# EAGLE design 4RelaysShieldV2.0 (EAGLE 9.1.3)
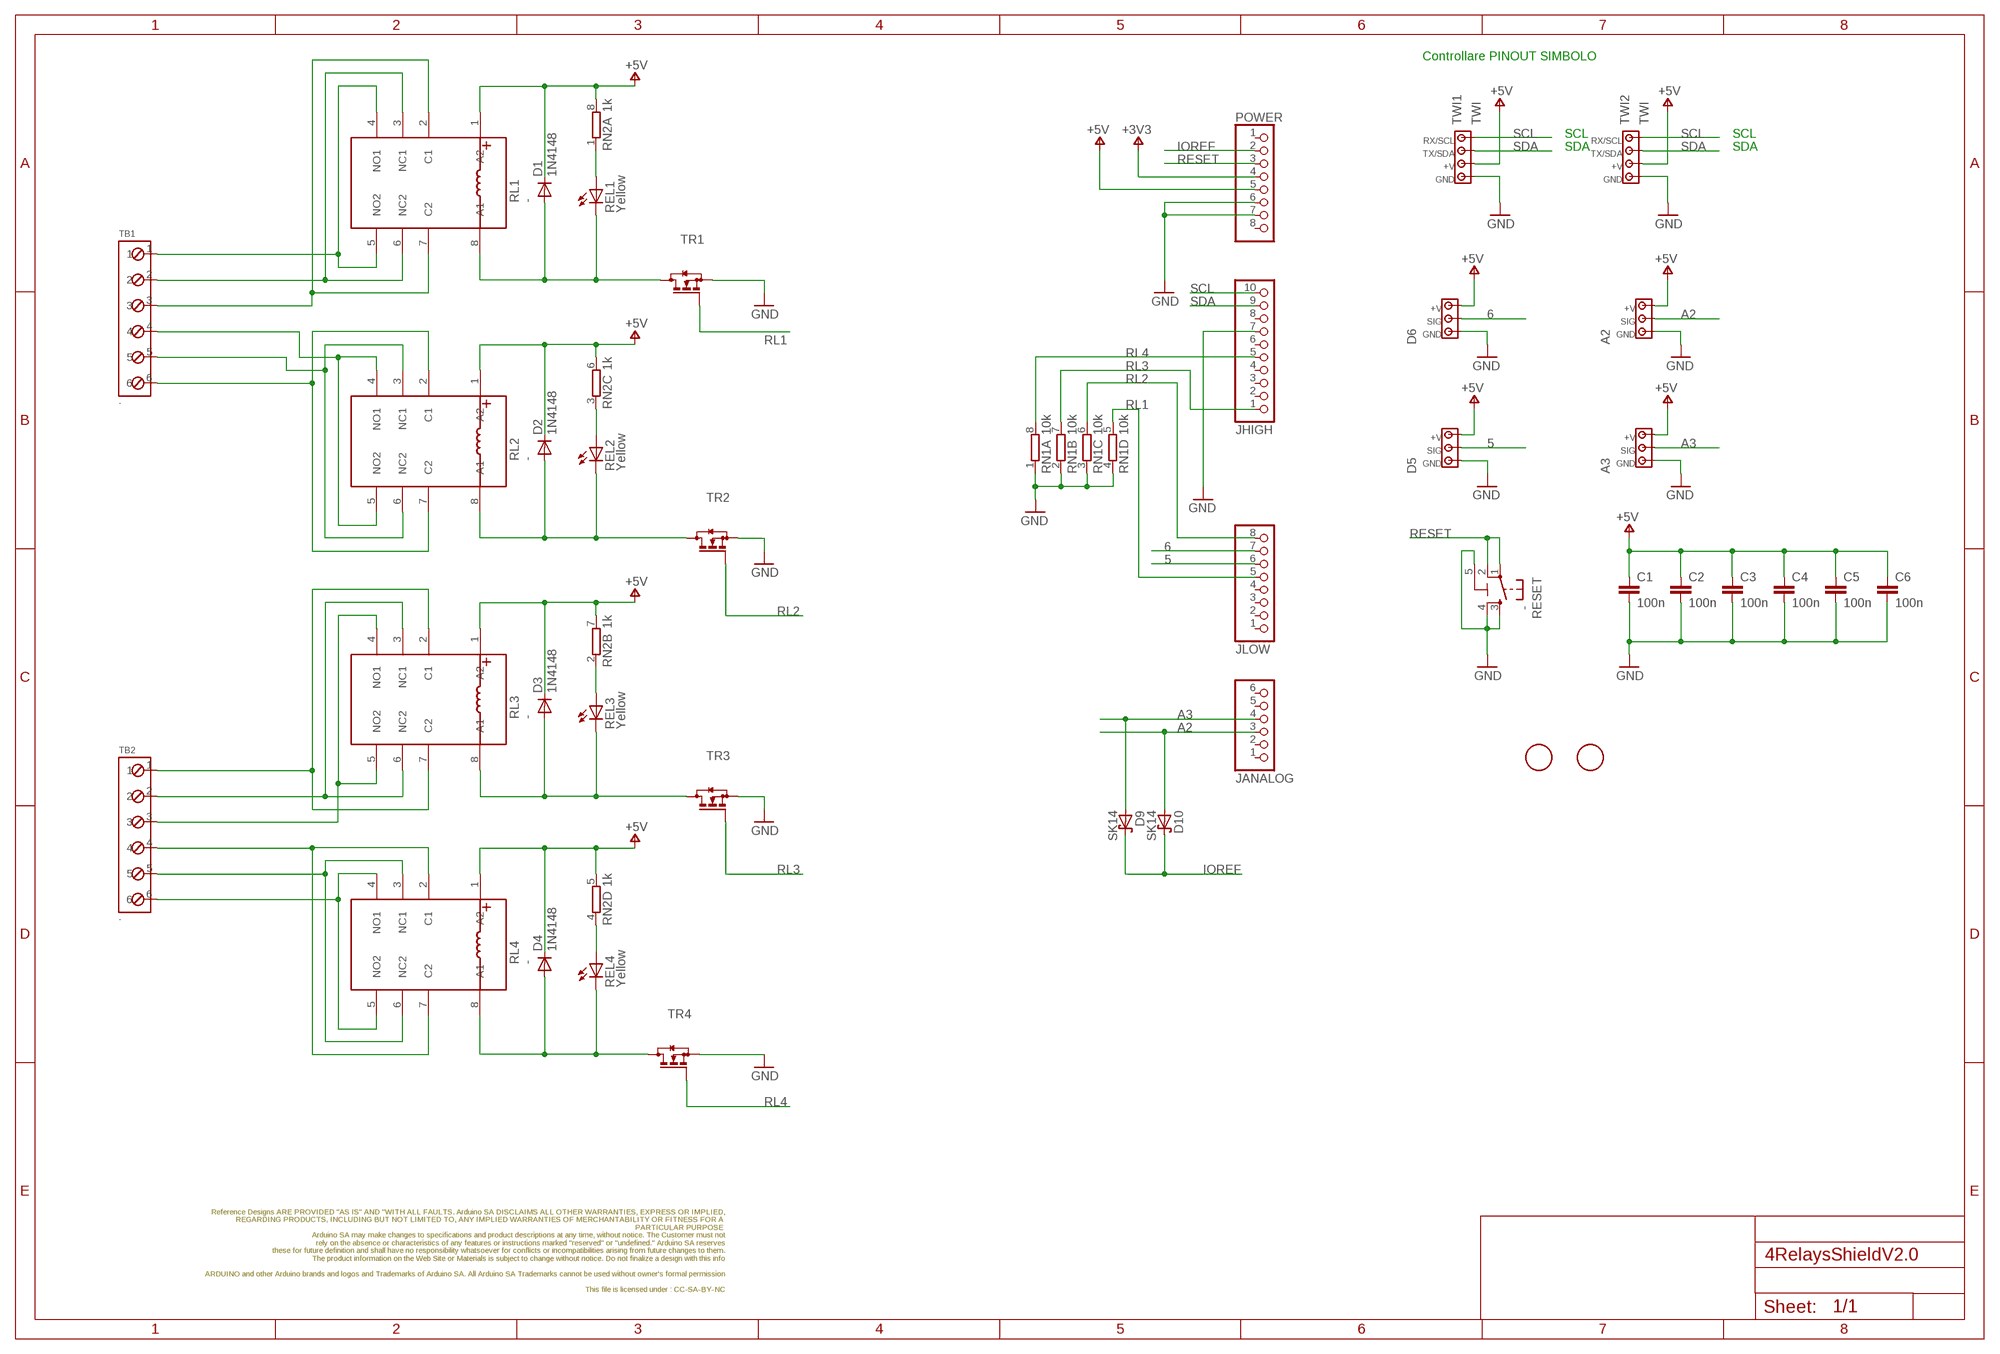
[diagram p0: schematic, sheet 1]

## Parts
A2  -  MODULINO-3-IN  [MODULINO-3]
A3  -  MODULINO-3-IN  [MODULINO-3]
C1  100n  C-100NF-0603  [0603-1608X90N]
C2  100n  C-100NF-0603  [0603-1608X90N]
C3  100n  C-100NF-0603  [0603-1608X90N]
C4  100n  C-100NF-0603  [0603-1608X90N]
C5  100n  C-100NF-0603  [0603-1608X90N]
C6  100n  C-100NF-0603  [0603-1608X90N]
D1  1N4148  DIODE-SOD123  [SOD123]
D2  1N4148  DIODE-SOD123  [SOD123]
D3  1N4148  DIODE-SOD123  [SOD123]
D4  1N4148  DIODE-SOD123  [SOD123]
D5  OUT  MODULINO-3-OUT  [MODULINO-3]
D6  OUT  MODULINO-3-OUT  [MODULINO-3]
D9  SK14  D_SCHOTTKY-SMB-SMB  [SMB_DO214AA]
D10  SK14  D_SCHOTTKY-SMB-SMB  [SMB_DO214AA]
FID2  DNP  FIDUCIAL-2MM  [FD-1-2]
FID3  DNP  FIDUCIAL-2MM  [FD-1-2]
FRAME1  A3-FRAMEONLY  [FRAME-NO-BAN-FRAMEONLY]
FRAME2  TEXTTEXT_BRDSCH  [FRAME]
JANALOG  Analog  PINHD-1X06TH  [1X06-TH]
JHIGH  Digital  PINHD-1X10TH  [1X10]
JLOW  Digital  PINHD-1X08-DIGITALTH  [1X08]
POWER  Power  PINHD-1X08-POWERTH  [1X08]
REL1  Yellow  0044_KPT-2012YC  [CHIPLED_0805]
REL2  Yellow  0044_KPT-2012YC  [CHIPLED_0805]
REL3  Yellow  0044_KPT-2012YC  [CHIPLED_0805]
REL4  Yellow  0044_KPT-2012YC  [CHIPLED_0805]
RESET  -  TACTILE2  [TS42]
RL1  -  RELAY-5  [RELE'-30SSERIES-DIL-2X]
RL2  -  RELAY-5  [RELE'-30SSERIES-DIL-2X]
RL3  -  RELAY-5  [RELE'-30SSERIES-DIL-2X]
RL4  -  RELAY-5  [RELE'-30SSERIES-DIL-2X]
RN1  10k  4R-N-10KCAY16  [CAY16]
RN2  1k  4R-N-1KCAY16  [CAY16]
TB1  -  0698_MRB316-3,81-V-BL  [MRB316-3,81-V-BL]
TB2  -  0698_MRB316-3,81-V-BL  [MRB316-3,81-V-BL]
TR1  2N7002  2N7002T-SOT23-SOT23  [SOT23]
TR2  2N7002  2N7002T-SOT23-SOT23  [SOT23]
TR3  2N7002  2N7002T-SOT23-SOT23  [SOT23]
TR4  2N7002  2N7002T-SOT23-SOT23  [SOT23]
TWI1  TWI  MODULINO-4-TWI  [MODULINO-4]
TWI2  TWI  MODULINO-4-TWI  [MODULINO-4]

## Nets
5: D5.2 JLOW.6
6: D6.2 JLOW.7
+3V3 [power]: POWER.4
+5V [power]: A2.1 A3.1 C1.1 C2.1 C3.1 C4.1 C5.1 C6.1 D1.C D2.C D3.C D4.C D5.1 D6.1 POWER.5 RL1.1(A2) RL2.1(A2) RL3.1(A2) RL4.1(A2) RN2.5 RN2.6 RN2.7 RN2.8 TWI1.3 TWI2.3
A2: A2.2 D10.A JANALOG.3
A3: A3.2 D9.A JANALOG.4
GND [power]: A2.3 A3.3 C1.2 C2.2 C3.2 C4.2 C5.2 C6.2 D5.3 D6.3 JHIGH.7 POWER.6 POWER.7 RESET.3 RESET.4 RESET.5(5-GND) RN1.1 RN1.2 RN1.3 RN1.4 TR1.2(S) TR2.2(S) TR3.2(S) TR4.2(S) TWI1.4 TWI2.4
IOREF: D9.C D10.C POWER.2
N$1: REL1.A RN2.1
N$2: REL2.A RN2.3
N$3: REL3.A RN2.2
N$4: REL4.A RN2.4
N$14: D1.A REL1.C RL1.8(A1) TR1.3(D)
N$16: D2.A REL2.C RL2.8(A1) TR2.3(D)
N$18: D3.A REL3.C RL3.8(A1) TR3.3(D)
N$20: D4.A REL4.C RL4.8(A1) TR4.3(D)
REL1_COM [RelayOut]: RL1.2(C1) RL1.7(C2) TB1.3
REL1_NC [RelayOut]: RL1.3(NC1) RL1.6(NC2) TB1.2
REL1_NO [RelayOut]: RL1.4(NO1) RL1.5(NO2) TB1.1
REL2_COM [RelayOut]: RL2.2(C1) RL2.7(C2) TB1.6
REL2_NC [RelayOut]: RL2.3(NC1) RL2.6(NC2) TB1.5
REL2_NO [RelayOut]: RL2.4(NO1) RL2.5(NO2) TB1.4
REL3_COM [RelayOut]: RL3.2(C1) RL3.7(C2) TB2.1
REL3_NC [RelayOut]: RL3.3(NC1) RL3.6(NC2) TB2.2
REL3_NO [RelayOut]: RL3.4(NO1) RL3.5(NO2) TB2.3
REL4_COM [RelayOut]: RL4.2(C1) RL4.7(C2) TB2.4
REL4_NC [RelayOut]: RL4.3(NC1) RL4.6(NC2) TB2.5
REL4_NO [RelayOut]: RL4.4(NO1) RL4.5(NO2) TB2.6
RESET: POWER.3 RESET.1 RESET.2
RL1: JLOW.5 RN1.5 TR1.1(G)
RL2: JLOW.8 RN1.6 TR2.1(G)
RL3: JHIGH.1 RN1.7 TR3.1(G)
RL4: JHIGH.5 RN1.8 TR4.1(G)
SCL: JHIGH.10 TWI1.1 TWI2.1
SDA: JHIGH.9 TWI1.2 TWI2.2
Unconnected: JANALOG.1 JANALOG.2 JANALOG.5 JANALOG.6 JHIGH.2 JHIGH.3 JHIGH.4 JHIGH.6 JHIGH.8 JLOW.1 JLOW.2 JLOW.3 JLOW.4 POWER.1 POWER.8

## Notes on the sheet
- Controllare PINOUT SIMBOLO
- SCL | SCL
- SDA | SDA

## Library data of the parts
A2 A3 = Arduino-connectors:MODULINO-3: Modulino 4 connector; CODE-BCE: SP1695; CODE-BCMI: 1695; CODE-TK2: -; DATASHEET: -; DISTRIBUTOR-LINK: -; DISTRIBUTOR-PN: -; MANUFACTURER: -; MANUFACTURER-PN: -
C1-C6 = Arduino-rcl:C: SMD Capacitor; CODE-ARDUINO: -; DATASHEET: http://search.murata.co.jp/Ceramy/image/img/A01X/G101/ENG/GRM188R71C104KA01-01.pdf; DISTRIBUTOR-LINK: https://www.digikey.com/product-detail/en/murata-electronics-north-america/GRM188R71C104KA01D/490-1532-1-ND/587771; DISTRIBUTOR-PN: 490-1532-2-ND; MANUFACTURER: Murata; MANUFACTURER-PN: GRM188R71C104KA01D; NOTE: -
D1-D4 = Arduino-diodes:DIODE: FAST SMALL SIGNAL DIODES SMD 200mA 100V SOD123; CODE-BCE: SP0234; CODE-BCMI: 0234; CODE-TK2: -; DATASHEET: http://www.mccsemi.com/up_pdf/1N4148WX(SOD323).pdf; DISTRIBUTOR-LINK: https://www.digikey.com/product-detail/it/micro-commercial-co/1N4148WX-TP/1N4148WXTPMSCT-ND/717312; DISTRIBUTOR-PN: 1N4148WXTPMSCT-ND; MANUFACTURER: Micro Commercial Co; MANUFACTURER-PN: 1N4148WX-TP
D5 D6 = Arduino-connectors:MODULINO-3: Modulino 4 connector; CODE-BCE: SP1696; CODE-BCMI: 1696; CODE-TK2: -; DATASHEET: -; DISTRIBUTOR-LINK: -; DISTRIBUTOR-PN: -; MANUFACTURER: -; MANUFACTURER-PN: -
D9 D10 = Arduino-diodes:D_SCHOTTKY: Schottky Diodes; CODE-ARDUINO: 0234; DATASHEET: http://www.mccsemi.com/up_pdf/SK12-L~SK110-L(DO-214AA).PDF; DISTRIBUTOR-LINK: https://www.digikey.com/product-detail/it/micro-commercial-co/SK14-LTP/SK14-LTPMSCT-ND/2642062; DISTRIBUTOR-PN: SK14-LTPMSCT-ND; MANUFACTURER: Micro Commercial Co; MANUFACTURER-PN: SK14-LTP
FID2 FID3 = Arduino-utility:FIDUCIAL: Fiducial mount; CODE-ARDUINO: DNP; DATASHEET: DNP; DISTRIBUTOR-LINK: DNP; DISTRIBUTOR-PN: DNP; MANUFACTURER: DNP; MANUFACTURER-PN: DNP
FRAME1 = Arduino-utility:A3-FRAMEONLY: Schematic frame
FRAME2 = Arduino-utility:TEXT: TEXT
JANALOG = Arduino-connectors:PINHD-1X06: PIN HEADER; CODE-ARDUINO: 3649; DATASHEET: -; DISTRIBUTOR-LINK: -; DISTRIBUTOR-PN: -; MANUFACTURER: -; MANUFACTURER-PN: FH254-106DF085149V
JHIGH = Arduino-connectors:PINHD-1X10: PIN HEADER; CODE-ARDUINO: 3648; DATASHEET: -; DISTRIBUTOR-LINK: -; DISTRIBUTOR-PN: -; MANUFACTURER: -; MANUFACTURER-PN: FH254-110DF085149V
JLOW = Arduino-connectors:PINHD-1X08: PIN HEADER; CODE-ARDUINO: 3648; DATASHEET: -; DISTRIBUTOR-LINK: -; DISTRIBUTOR-PN: -; MANUFACTURER: -; MANUFACTURER-PN: FH254-108DF085149V
POWER = Arduino-connectors:PINHD-1X08: PIN HEADER; CODE-ARDUINO: 3649; DATASHEET: -; DISTRIBUTOR-LINK: -; DISTRIBUTOR-PN: -; MANUFACTURER: -; MANUFACTURER-PN: FH254-108DF085149V
REL1-REL4 = Opto:0044_KPT-2012YC: LED YELLOW - SMD - 0805; MONTHLY_USAGE: _____; PART_NUMBER: KPT-2012YC; PRICE: _____; SUPPLIER: _____; TYPE: Opto
RESET = Arduino-pushbuttons:TACTILE2: Pushbutton; CODE-ARDUINO: 0946; DATASHEET: http://www.mouser.com/ds/2/418/NG_CD_1571636_C1-122399.pdf; DISTRIBUTOR-LINK: https://www.mouser.it/ProductDetail/TE-Connectivity/1571636-3/?qs=%2fha2pyFaduiys%2fNUBzym%252bcoSb9tuK3Sjuv54qjf0hQ0%3d; DISTRIBUTOR-PN: 506-1571636-3; MANUFACTURER: TE; MANUFACTURER-PN: 1571636-3
RL1-RL4 = Arduino-mechanical:RELAY-5: Relay 5V black Omron; CODE-BCE: SP0773; CODE-BCMI: 0773; CODE-TK2: -; DATASHEET: http://omronfs.omron.com/en_US/ecb/products/pdf/en-g5v_2.pdf; DISTRIBUTOR-LINK: https://www.digikey.com/product-detail/it/omron-electronics-inc-emc-div/G5V-2-H1-DC5/Z108-ND/277844; DISTRIBUTOR-PN: Z108-ND; MANUFACTURER: Omron; MANUFACTURER-PN: G5V-2-H1 DC5
RN1 = Arduino-rcl:4R-N: Array Chip Resistor Source: RS Component / Phycomp; CODE-ARDUINO: 0016; DATASHEET: http://www.bourns.com/docs/Product-Datasheets/CATCAY.pdf; DISTRIBUTOR-LINK: https://www.digikey.com/products/en?keywords=CAY16-103J4LFTR-ND; DISTRIBUTOR-PN: CAY16-103J4LFTR-ND; MANUFACTURER: Bourns Inc.; MANUFACTURER-PN: CAY16-103J4LF; RESTRICTIONS: NO
RN2 = Arduino-rcl:4R-N: Array Chip Resistor Source: RS Component / Phycomp; CODE-ARDUINO: 0005; DATASHEET: http://www.bourns.com/docs/Product-Datasheets/CATCAY.pdf; DISTRIBUTOR-LINK: https://www.digikey.com/product-detail/en/bourns-inc/CAY16-102J4LF/CAY16-102J4LFCT-ND/3437828; DISTRIBUTOR-PN: CAY16-102J4LFCT-ND; MANUFACTURER: Bourns Inc.; MANUFACTURER-PN: CAY16-102J4LF; RESTRICTIONS: NO
TB1 TB2 = Arduino-connectors:0698_MRB316-3,81-V-BL: Morsetto 6 poli h8,5mm Blue - EURO-BLOCK; CODE-BCE: SP0698; CODE-BCMI: 0698; CODE-TK2: -; DATASHEET: -; DISTRIBUTOR-LINK: -; DISTRIBUTOR-PN: -; MANUFACTURER: -; MANUFACTURER-PN: MRB316-3,81-V-BL
TR1-TR4 = Arduino-transistors:2N7002T: MOSFET N-CH 60V 115MA; CODE-ARDUINO: -; DATASHEET: http://www.mccsemi.com/up_pdf/2N7002(SOT-23).PDF; DISTRIBUTOR-LINK: https://www.digikey.com/product-detail/it/micro-commercial-co/2N7002-TP/2N7002-TPMSCT-ND/1960099; DISTRIBUTOR-PN: 2N7002-TPMSCT-ND; MANUFACTURER: Micro Commercial Co; MANUFACTURER-PN: 2N7002-TP
TWI1 TWI2 = Arduino-connectors:MODULINO-4: Modulino 4 connector; CODE-BCE: SP1693; CODE-BCMI: 1693; CODE-TK2: -; DATASHEET: -; DISTRIBUTOR-LINK: -; DISTRIBUTOR-PN: -; MANUFACTURER: -; MANUFACTURER-PN: -

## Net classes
0 default: width 0.254 mm, drill 0.61 mm, clearance 0.152 mm
1 power: width 0.305 mm, drill 0.61 mm, clearance 0.305 mm
2 VIN: width 0.305 mm, drill 0.61 mm, clearance 0.152 mm
3 RelayOut: width 1.27 mm, clearance 4 mm to class 0, clearance 4 mm to class 1, clearance 4 mm to class 2, clearance 1.27 mm

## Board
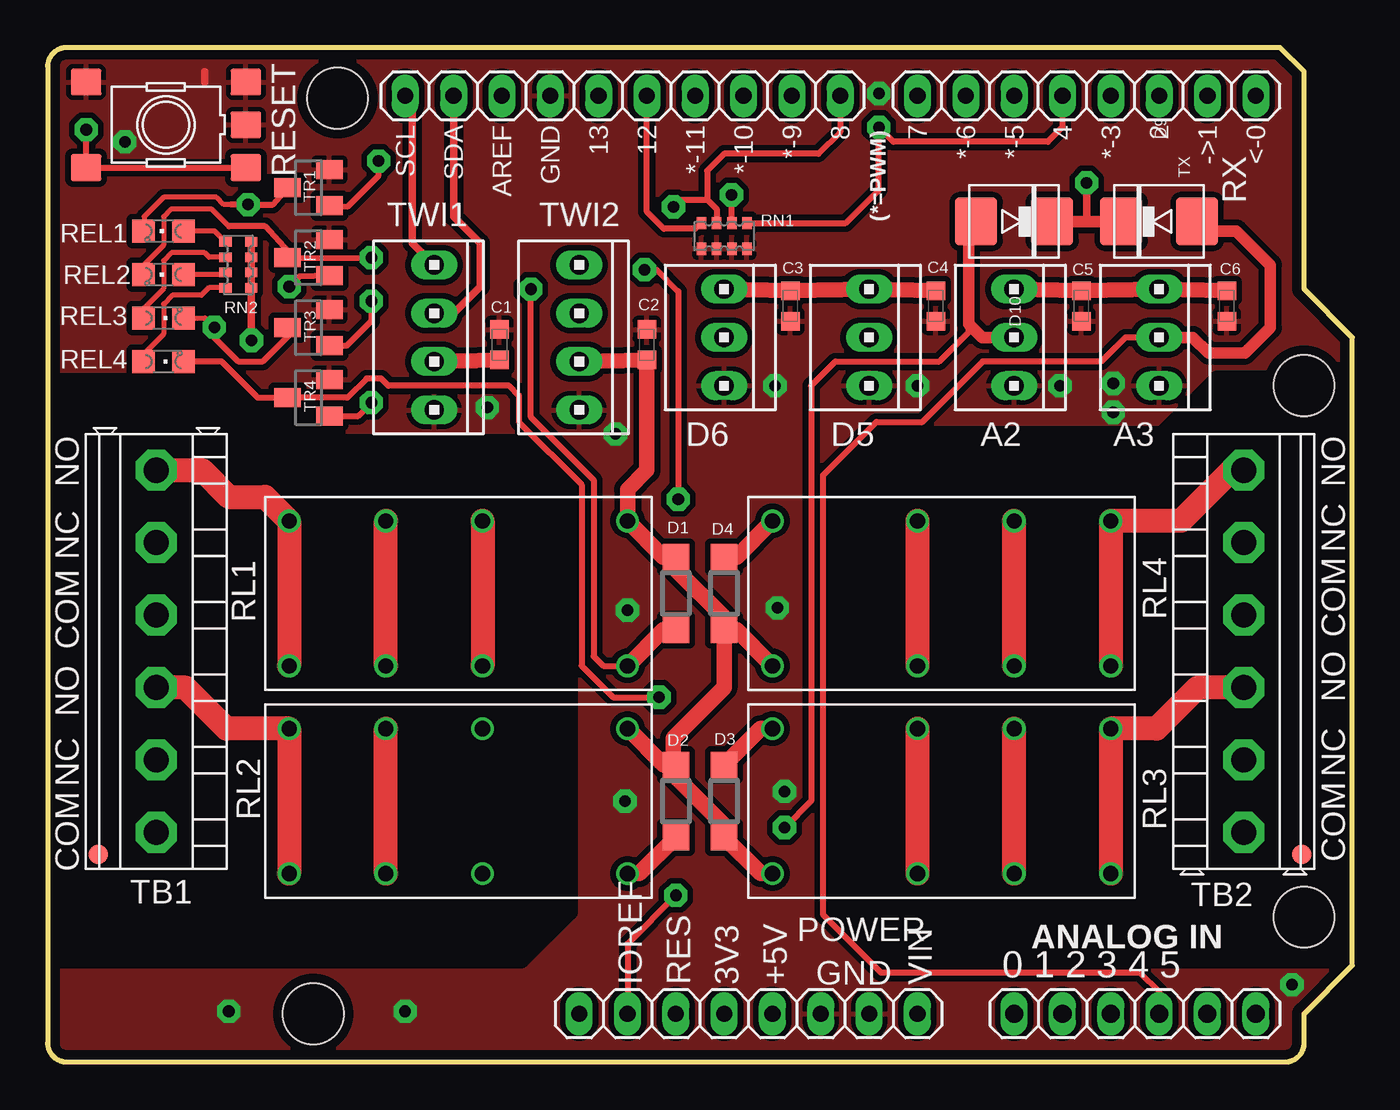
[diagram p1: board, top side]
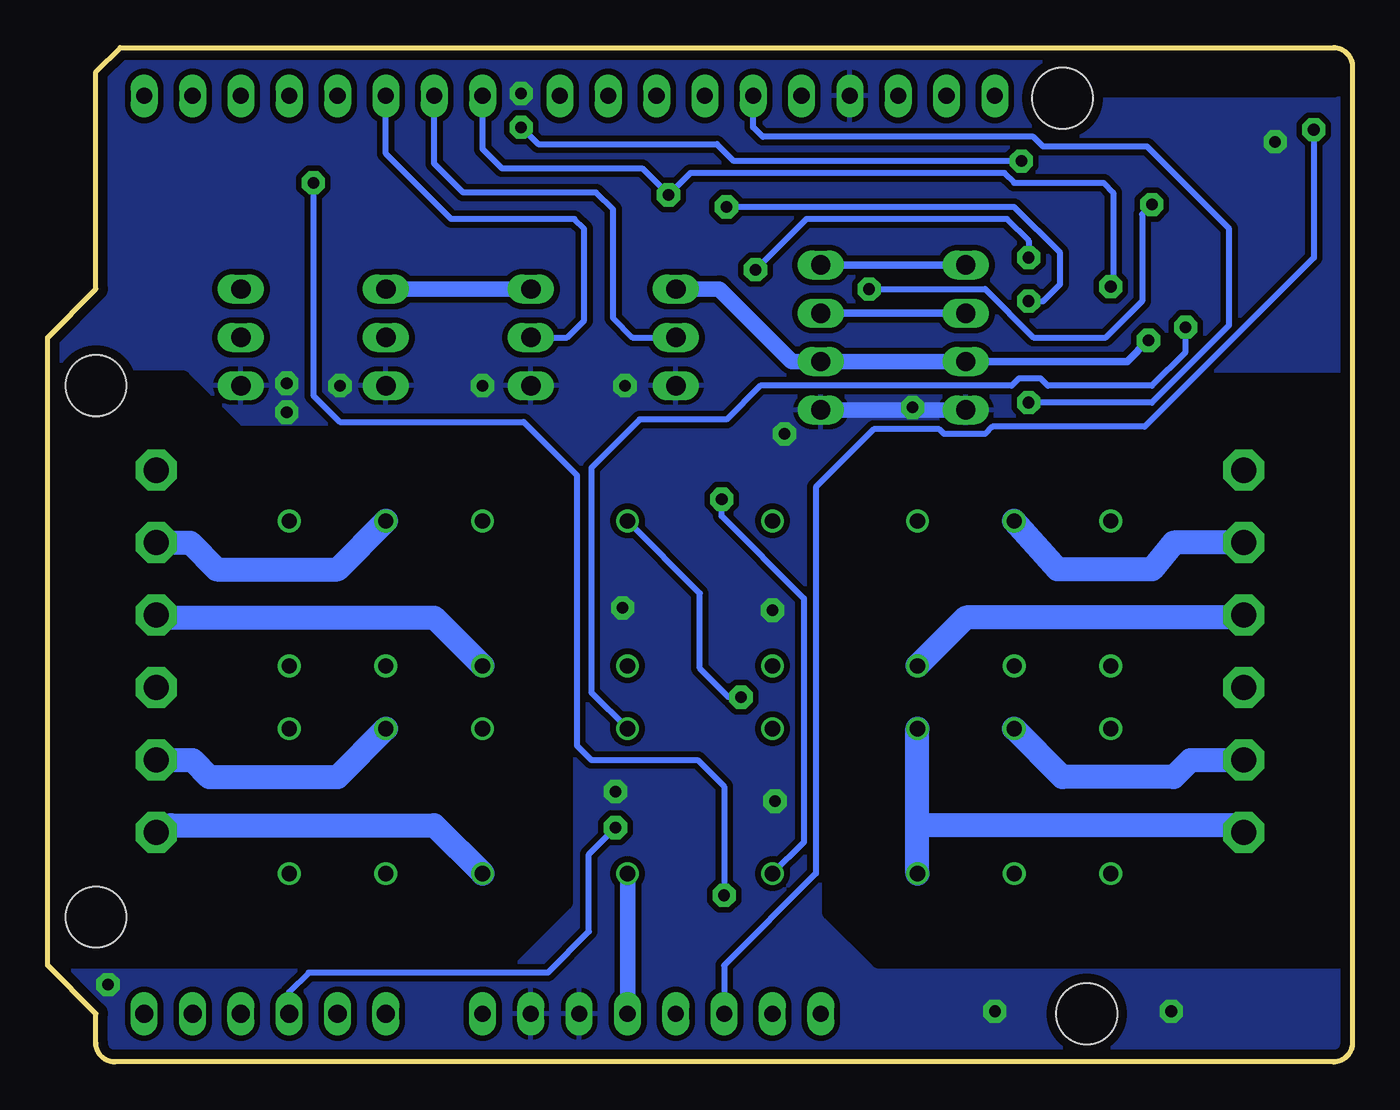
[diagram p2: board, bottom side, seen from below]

Size 68.58 x 53.34 mm. Coordinates in mm from the lower left corner, seen from the top.
Outline: 66.04,2.54 68.58,5.08 68.58,38.1 66.04,40.64 66.04,52.07 64.77,53.34 1,53.34 arc90 0,52.34 0,1 arc90 1,0 65.04,0 arc90 66.04,1 66.04,2.54
Copper layers (1*16): Top 0.035mm / dielectric 1.5mm / Bottom 0.035mm
Design rules "default *": minimum track width 10mil, minimum drill 10mil, track to track 12mil, track to pad 12mil, pad to pad 12mil, via to via 12mil, smd to smd 12mil, copper to edge 20mil, drill to drill 10mil, minimum pad ring 6mil, minimum via ring 12mil, stop-mask expansion 2mil, vias tented up to drill 32mil, thermal gap 10mil
Holes 3.2 mm at 66.04,35.56 66.04,7.62 15.24,50.67 13.97,2.54
tRestrict: 18 lines
bRestrict: 21 lines

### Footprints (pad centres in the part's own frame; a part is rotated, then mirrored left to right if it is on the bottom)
MODULINO-3 = drill 1.016 long: 1 -2.54,0; 2 0,0; 3 2.54,0
0603-1608X90N = smd 0.95 x 1: 1 -0.8,0; 2 0.8,0
SOD123 = smd 1.4 x 1.4: A 1.9,0; C -1.9,0
SMB_DO214AA = smd 2.5 x 2.2: A 0,-2; C 0,2
FD-1-2 = smd 1.016 x 1.016: P$1 0,0
1X06-TH = drill 0.95 pad 1.422 long: 1 -6.35,0; 2 -3.81,0; 3 -1.27,0; 4 1.27,0; 5 3.81,0; 6 6.35,0
1X10 = drill 0.85 pad 1.422 long: 1 -11.43,0; 2 -8.89,0; 3 -6.35,0; 4 -3.81,0; 5 -1.27,0; 6 1.27,0; 7 3.81,0; 8 6.35,0; 9 8.89,0; 10 11.43,0
1X08 = drill 0.85 pad 1.422 long: 1 -8.89,0; 2 -6.35,0; 3 -3.81,0; 4 -1.27,0; 5 1.27,0; 6 3.81,0; 7 6.35,0; 8 8.89,0
CHIPLED_0805 = smd 1.2 x 1.2: A 0,-1.05; C 0,1.05
TS42 = smd 1.6 x 1.4: 1 -4.2,2.25; 2 4.2,2.25; 3 -4.2,-2.25; 4 4.2,-2.25; 5 -4.2,0
RELE'-30SSERIES-DIL-2X = drill 0.8: 1 -7.62,-3.81; 2 0,-3.81; 3 5.08,-3.81; 4 10.16,-3.81; 5 10.16,3.81; 6 5.08,3.81; 7 0,3.81; 8 -7.62,3.81
CAY16 = smd 0.5 x 0.65: 1 -1.2,-0.675; 2 -0.4,-0.675; 3 0.4,-0.675; 4 1.2,-0.675; 5 1.2,0.675; 6 0.4,0.675; 7 -0.4,0.675; 8 -1.2,0.675
MRB316-3,81-V-BL = drill 1.321 pad 2.159 octagon: 1 0,9.525; 2 0,5.715; 3 0,1.905; 4 0,-1.905; 5 0,-5.715; 6 0,-9.525
SOT23 = smd 1 x 1.4: 1 -0.95,-1.1; 2 0.95,-1.1; 3 0,1.1
MODULINO-4 = drill 1.016 long: 1 3.81,0; 2 1.27,0; 3 -1.27,0; 4 -3.81,0

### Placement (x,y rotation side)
A2  50.8,38.1 270 top
A3  58.42,38.1 270 top
C1  23.75,37.72 90 top
C2  31.5,37.72 90 top
C3  39.04,39.75 270 top
C4  46.69,39.75 270 top
C5  54.33,39.75 270 top
C6  61.98,39.75 270 top
D1  33.02,24.64 270 top
D2  33.02,13.72 270 top
D3  35.56,13.72 90 top
D4  35.56,24.64 90 top
D5  43.18,38.1 270 top
D6  35.56,38.1 270 top
D9  58.42,44.2 90 top
D10  50.8,44.2 270 top
FID2  2.67,10.92 0 top
FID3  65.91,10.92 0 top
FRAME1  -0.13,-0.25 0 top
FRAME2  not placed on the board
JANALOG  57.15,2.54 0 top
JHIGH  30.23,50.8 180 top
JLOW  54.61,50.8 180 top
POWER  36.83,2.54 0 top
REL1  6.1,43.69 90 top
REL2  6.1,41.4 90 top
REL3  6.1,39.12 270 top
REL4  6.1,36.83 270 top
RESET  6.22,49.28 180 top
RL1  22.86,24.64 180 top
RL2  22.86,13.72 180 top
RL3  45.72,13.72 0 top
RL4  45.72,24.64 0 top
RN1  35.56,43.43 0 top
RN2  10.03,41.91 270 top
TB1  5.71,21.59 0 top
TB2  62.87,21.59 180 top
TR1  13.72,45.97 90 top
TR2  13.72,42.29 90 top
TR3  13.72,38.61 90 top
TR4  13.72,34.92 90 top
TWI1  20.32,38.1 90 top
TWI2  27.94,38.1 90 top

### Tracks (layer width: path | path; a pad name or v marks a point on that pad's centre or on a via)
5
  Bottom 0.305: D5.2 41.27,38.1 40.39,38.99 40.39,43.81 40.89,44.32 47.37,44.32 50.8,47.75 JLOW.6
6
  Bottom 0.305: D6.2 37.85,38.1 38.86,39.12 38.86,44.83 39.75,45.72 46.74,45.72 48.26,47.24 JLOW.7
+5V  (via drill 0.61)
  Top 0.406: v10.72,37.95 10.71,37.96 RN2.5 RN2.6 RN2.7 RN2.8
  Top 0.813: D6.1 C3.1 D5.1 C4.1 | A2.1 C5.1 A3.1 C6.1 | TWI2.3 C2.1 31.5,31.11 30.48,30.1 RL1.1 32.39,26.54 D1.C 33.02,25.91 35.56,23.37 D4.C | C1.1 TWI1.3 | D4.C 36.19,22.74 RL4.1 | RL3.1 37.47,9.91 D3.C 35.56,12.45 33.02,14.99 D2.C | D2.C 32.39,15.62 RL2.1 | D4.C 35.56,19.68 32.89,17.02 32.89,15.74 D2.C
  Bottom 0.406: TWI1.3 11.84,36.83 v10.72,37.95
  Bottom 0.813: TWI1.3 TWI2.3 29.46,36.83 33.27,40.64 D6.1 | RL3.1 POWER.5 | A2.1 D5.1
A2  (via drill 0.61)
  Top 0.305: v38.73,12.32 40.13,13.72 40.13,35.56 41.4,36.83 46.86,36.83 48.41,38.38 48.41,39.12
  Top 0.61: A2.2 49.12,38.1 48.41,38.81 48.41,39.12 48.41,44.2 D10.A
  Bottom 0.305: v38.73,12.32 40.13,10.92 40.13,6.86 42.29,4.7 54.86,4.7 55.88,3.68 JANALOG.3
A3
  Top 0.305: A3.2 56.64,38.1 55.37,36.83 49.15,36.83 45.97,33.66 43.56,33.66 40.77,30.86 40.77,7.75 43.81,4.7 57.4,4.7 58.42,3.68 JANALOG.4
  Top 0.61: A3.2 60.2,38.1 61.04,37.26 62.92,37.26 64.26,38.61 64.26,41.91 62.48,43.69 61.13,43.69 D9.A
GND  (via drill 0.61)
  Top 0.406: 8.26,52.07 8.26,51.53
  Bottom 0.813: TWI1.4 TWI2.4
  other vias: 43.69,50.93 65.41,4.06 38.73,14.22 18.8,2.67 4.06,48.39 9.53,2.67 23.11,34.42 29.84,33.02 38.23,35.56 45.72,35.56 53.21,35.56 56.01,35.69 56.01,34.16 30.48,23.75 38.35,23.88 30.35,13.72
  pour Bottom (isolate 0.305): 0,53.34 68.58,53.34 68.58,0 0,0
  pour Top (isolate 0.305): 0,53.34 68.58,53.34 68.58,0 0,0
IOREF  (via drill 0.61)
  Top 0.305: v33.02,8.76 30.48,6.22 POWER.2
  Top 0.406: v54.61,46.23 54.61,44.2
  Top 0.61: D10.C 54.61,44.2 D9.C
  Bottom 0.305: v54.61,46.23 54.61,35.05 53.21,33.66 43.56,33.66 40.77,30.86 40.77,16.64 40.01,15.88 34.42,15.88 33.02,14.48 v33.02,8.76
N$1
  Top 0.254: RN2.1 8.78,43.69 REL1.A
N$2
  Top 0.254: RN2.3 9.25,41.4 REL2.A
N$3
  Top 0.254: RN2.2 8.49,42.31 8.26,42.55 6.5,42.55 6.1,42.14 6.1,40.66 5.05,39.62 REL3.A
N$4
  Top 0.254: RN2.4 8.48,40.71 8.08,40.31 6.55,40.31 6.1,39.85 6.1,38.28 5.05,37.23 REL4.A
N$14  (via drill 0.61)
  Top 0.254: 9.65,45.09 9.27,45.09 8.89,45.47 6.1,45.47 5.08,44.45 5.08,43.42 REL1.C
  Top 0.305: TR1.3 11.84,45.09 v10.54,45.09 9.65,45.09 | v25.4,40.64 25.4,33.91 28.7,30.61 28.7,21.34 29.21,20.83 RL1.8
  Top 0.813: D1.A 32.39,22.74 RL1.8
  Bottom 0.305: v25.4,40.64 19.3,40.64 16.76,38.1 12.95,38.1 11.05,40.01 11.05,44.58 v10.54,45.09
N$16  (via drill 0.61)
  Top 0.254: 9.53,43.94 8.64,44.83 6.48,44.83 6.1,44.45 6.1,42.95 5.05,41.9 REL2.C
  Top 0.305: v31.37,41.66 32,41.66 33.15,40.51 v33.15,29.59 | v17.02,42.29 16.99,42.26 TR2.3 12.68,42.29 12.68,42.57 11.43,43.94 9.53,43.94
  Top 0.813: RL2.8 31.11,9.91 D2.A
  Bottom 0.305: v31.37,41.66 28.7,44.32 18.16,44.32 17.02,43.18 v17.02,42.29 | v33.15,29.59 33.15,28.7 28.83,24.38 28.83,11.56 RL2.8
N$18  (via drill 0.61)
  Top 0.254: REL3.C 8.28,39.12 v8.76,38.63
  Top 0.305: v8.76,38.63 8.76,38.1 10.03,36.83 11.3,36.83 12.7,38.23 TR3.3
  Top 0.813: RL3.8 37.47,17.53 D3.A
  Bottom 0.305: RL3.8 40.01,19.43 40.01,31.24 37.47,33.78 32.89,33.78 31.11,35.56 17.91,35.56 17.53,35.94 16.38,35.94 16,35.56 10.54,35.56 8.76,37.34 v8.76,38.63
N$20  (via drill 0.61)
  Top 0.305: v32.13,19.18 29.72,19.18 28.07,20.83 28.07,30.35 24.77,33.66 24.77,35.05 24.26,35.56 17.91,35.56 17.53,35.94 16.76,35.94 15.75,34.92 TR4.3 11.05,34.92 9.14,36.83 REL4.C
  Top 0.813: D4.A 36.19,26.54 RL4.8
  Bottom 0.305: RL4.8 34.29,24.64 34.29,20.7 32.77,19.18 v32.13,19.18
REL1_COM
  Top 1.27: RL1.2 RL1.7
  Bottom 1.27: TB1.3 5.84,23.37 20.32,23.37 RL1.7
REL1_NC
  Top 1.27: RL1.6 RL1.3
  Bottom 1.27: TB1.2 9.4,27.3 10.54,25.91 15.49,25.91 RL1.3
REL1_NO
  Top 1.27: RL1.5 RL1.4 11.43,29.72 9.53,29.72 8.13,31.11 TB1.1
REL2_COM
  Bottom 1.27: RL2.7 22.86,12.45 | 22.86,12.45 RL2.2 | 22.86,12.45 6.1,12.45 TB1.6
REL2_NC
  Top 1.27: RL2.6 RL2.3
  Bottom 1.27: TB1.5 8.51,15.88 9.4,14.99 15.24,14.99 RL2.3
REL2_NO
  Top 1.27: RL2.5 RL2.4 9.4,17.53 7.24,19.68 TB1.4
REL3_COM
  Top 1.27: RL3.7 RL3.2
  Bottom 1.27: TB2.1 62.48,12.06 62.1,12.45 48.26,12.45 RL3.2
REL3_NC
  Top 1.27: RL3.3 RL3.6
  Bottom 1.27: TB2.2 60.96,15.88 60.07,14.99 53.34,14.99 RL3.6
REL3_NO
  Top 1.27: TB2.3 60.45,19.68 58.29,17.53 RL3.5 RL3.4
REL4_COM
  Top 1.27: RL4.7 RL4.2
  Bottom 1.27: RL4.2 48.26,23.37 62.74,23.37 TB2.4
REL4_NC
  Top 1.27: RL4.3 RL4.6
  Bottom 1.27: TB2.5 61.09,27.3 59.69,25.91 53.34,25.91 RL4.6
REL4_NO
  Top 1.27: TB2.6 62.23,31.11 59.56,28.45 RL4.5 RL4.4
RESET  (via drill 0.61)
  Top 0.305: v2.03,49.02 v2.02,49.01 RESET.2 RESET.1
  Bottom 0.305: v2.03,49.02 2.03,42.29 10.92,33.4 18.92,33.4 19.3,33.02 21.46,33.02 21.72,33.27 25.15,33.27 28.19,30.23 28.19,9.91 33.02,5.08 POWER.3
RL1  (via drill 0.61)
  Top 0.305: TR1.1 15.77,44.98 17.4,46.61 v17.4,47.37 | JLOW.5 53.34,49.15 52.58,48.39 44.45,48.39 v43.69,49.15 43.69,45.85 41.95,44.11 RN1.5
  Bottom 0.305: v17.4,47.37 32.51,47.37 33.4,48.26 42.8,48.26 v43.69,49.15
RL2  (via drill 0.61)
  Top 0.305: RN1.6 35.96,45.57 v35.94,45.59 | TR2.1 13.23,41.3 v12.7,40.77
  Bottom 0.305: v12.7,40.77 12.57,40.89 12.57,45.72 13.08,46.23 17.78,46.23 18.29,46.74 34.8,46.74 v35.94,45.59 37.34,46.99 44.7,46.99 45.72,48.01 JLOW.8
RL3  (via drill 0.61)
  Top 0.305: v17.02,40.01 17.02,38.96 15.7,37.64 14.76,37.64 TR3.1 | JHIGH.1 41.66,48.9 40.51,47.75 35.56,47.75 34.67,46.86 34.67,45.34 | 34.67,45.34 35.18,44.83 35.18,44.13 RN1.7 | v32.89,44.96 33.27,45.34 34.67,45.34
  Bottom 0.305: v17.02,40.01 16.26,40.01 15.37,40.89 15.37,42.55 17.78,44.96 v32.89,44.96
RL4  (via drill 0.61)
  Top 0.305: RN1.8 34.33,44.11 34.04,43.81 32.38,43.81 31.5,44.7 JHIGH.5 | TR4.1 16.32,33.98 v17.02,34.67
  Bottom 0.305: v17.02,34.67 10.54,34.67 6.48,38.73 6.48,43.81 10.79,48.13 16.26,48.13 16.76,48.64 30.99,48.64 31.5,49.15 JHIGH.5
SCL
  Top 0.406: JHIGH.10 19.18,50.42 19.18,43.05 TWI1.1
  Bottom 0.406: TWI1.1 TWI2.1
SDA
  Top 0.406: JHIGH.9 21.34,44.45 22.73,43.05 22.73,40.77 21.34,39.37 TWI1.2
  Bottom 0.406: TWI1.2 TWI2.2

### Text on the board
tNames: SCL | SDA | AREF | GND | 13 | 12 | *-11 | *-10 | *-9 | 8 | 7 | *-6 | *-5 | 4 | *-3 | 2 | ->1 | <-0 | TX | RX | (*=PWM) | NO | NO | NC | NC | COM | COM | NO | NO | NC | NC | COM | COM | ANALOG IN | IOREF | RES | 3V3 | +5V | GND | VIN | 0 1 2 3 4 5

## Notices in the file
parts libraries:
Arduino-utility: Copyright (c) 2016-2017 Arduino LLC. All right reserved.
Arduino-utility: This file is licensed under : CC-SA-BY-NC
